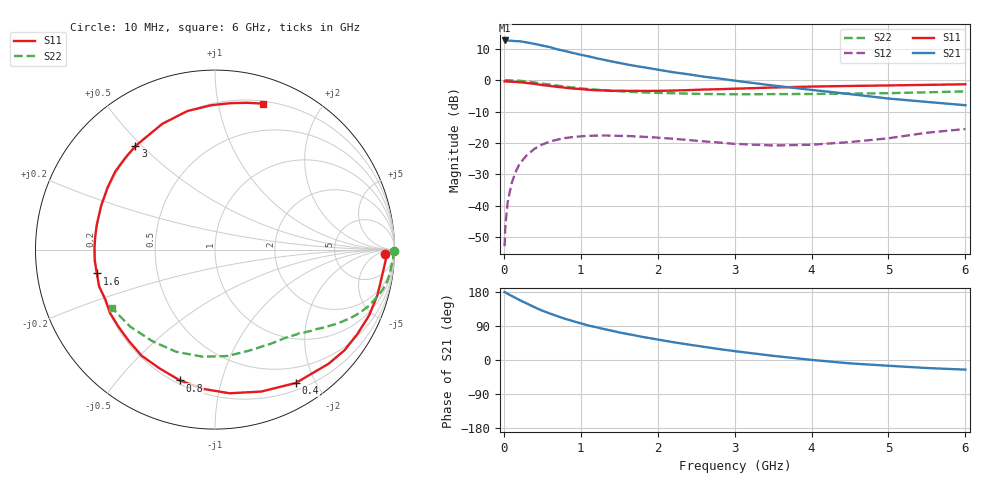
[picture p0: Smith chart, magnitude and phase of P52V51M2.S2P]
! SIEMENS Small Signal Semiconductors
! BFP183
! Si NPN RF Bipolar Junction Transistor in SOT143
! VCE = 2.5 V  IC = 1.2 mA
! Common Emitter S-Parameters:  March  1996
# GHz  S  MA  R  50
!  f  S11  S21  S12  S22
! GHz  MAG  ANG  MAG  ANG  MAG  ANG  MAG  ANG
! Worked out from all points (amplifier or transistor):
!   36 points, 10 MHz to 6 GHz, reference 50 ohm
!   highest |S21| = 12.6 dB at 10 MHz (marker M1)
!   |S21| within 3 dB of that: start of sweep to 727.9 MHz
!   unconditionally stable (mu >= 1): 2.394 GHz to end of sweep
!   at 250 MHz: K = 0.10, MSG = 18.7 dB, |S12| = -25.3 dB
!   at 1.4 GHz: K = 0.57, MSG = 11.8 dB, |S12| = -17.7 dB
!   at 6 GHz: K = 1.03, MAG = 2.7 dB, |S12| = -15.6 dB
!   S11 on the Smith chart (normalised r, x): 10 MHz: 31, -16; 400 MHz: 0.29, -1.74; 800 MHz: 0.22, -0.74; 1.6 GHz: 0.20, -0.10; 3 GHz: 0.19, +0.48; 6 GHz: 0.22, +1.35
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0.01  0.9497 -1.5  4.248 179.2  0.0023 90.0  0.9994 -0.5
0.02  0.9537 -3.2  4.245 178.6  0.0049 87.8  0.9912 -1.1
0.05  0.944 -7.7  4.24 174.7  0.0115 86.5  0.9944 -2.7
0.1  0.94 -15.5  4.197 169.4  0.0228 81.0  0.9867 -5.5
0.2  0.9224 -30.6  4.14 158.7  0.0454 72.0  0.9744 -10.8
0.25  0.9139 -37.9  4.043 153.6  0.0546 67.9  0.9607 -13.4
0.4  0.8688 -58.8  3.749 139.1  0.081 56.0  0.9147 -19.9
0.5  0.832 -71.9  3.528 130.2  0.0948 48.4  0.8788 -23.7
0.6  0.8045 -84.2  3.325 122.6  0.1058 42.5  0.8447 -26.9
0.7  0.7791 -94.7  3.059 115.4  0.1133 37.0  0.8121 -29.7
0.8  0.7545 -105.0  2.878 108.6  0.1199 32.0  0.7851 -32.1
0.9  0.7306 -114.9  2.687 102.5  0.1245 27.5  0.7599 -34.2
1.1  0.6998 -133.2  2.377 91.1  0.1299 19.9  0.7176 -38.1
1.3  0.6834 -148.8  2.094 81.8  0.1314 13.7  0.6886 -41.6
1.6  0.6715 -168.6  1.767 68.9  0.1293 6.7  0.6555 -46.1
1.8  0.6715 179.0  1.606 61.0  0.1257 3.5  0.6373 -49.3
2.2  0.6798 158.9  1.33 47.1  0.1168 -1.3  0.6165 -56.1
3  0.7279 127.5  0.977 23.4  0.0969 -1.2  0.5937 -72.1
3.5  0.7599 112.7  0.818 11.0  0.0913 5.4  0.5969 -83.3
4.5  0.8046 91.5  0.598 -8.9  0.1034 20.8  0.6091 -110.8
5.5  0.8378 77.5  0.449 -21.2  0.1456 25.4  0.6383 -137.7
6  0.8555 71.9  0.398 -25.4  0.1668 22.4  0.6597 -150.5
